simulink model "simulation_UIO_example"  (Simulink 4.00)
settings: Solver=VariableStepDiscrete  StartTime=0.0  StopTime=ts  RelTol=1e-3
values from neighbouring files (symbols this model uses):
  A = [0.9944 -0.1203 -0.4302    [UIO_example1.m]
  Ao = A - Ko*C    [UIO_example1.m]
  Auio = F    [UIO_example1.m]
  B = [0.4252 -0.0082 0.1813]'    [UIO_example1.m]
  Bo = [B Ko]    [UIO_example1.m]
  Buio = [T*B K]    [UIO_example1.m]
  C = eye(3)    [UIO_example1.m]
  Co = C    [UIO_example1.m]
  Cuio = C    [UIO_example1.m]
  D = zeros(3,3)    [UIO_example1.m]
  Do = zeros(3,4)    [UIO_example1.m]
  Duio = [zeros(3,1) H]    [UIO_example1.m]
  Tc = 0.1    [UIO_example1.m]
  x0 = [0.01 0.02 0.03]    [UIO_example1.m]

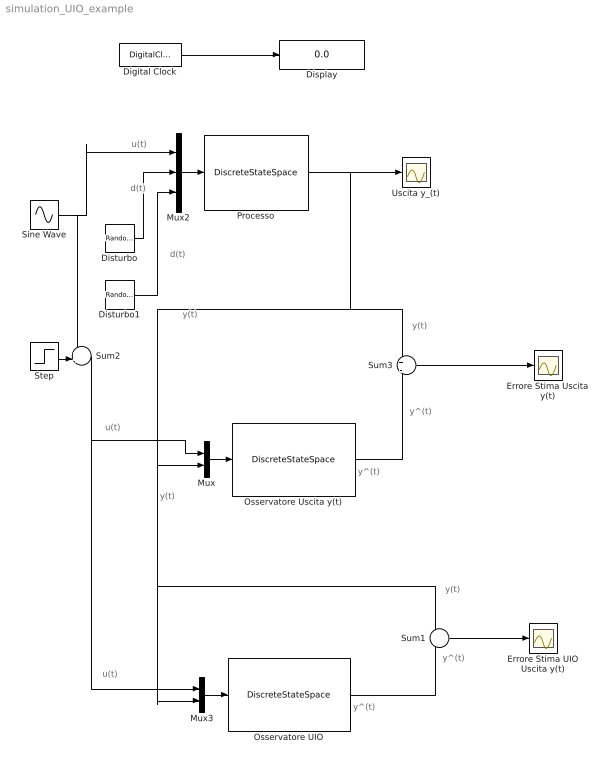
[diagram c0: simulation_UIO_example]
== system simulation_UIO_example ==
  note: d(t)
  note: u(t)
  note: y^(t)
  note: y(t)
  note: y^(t)
  note: y^(t)
  note: y^(t)
  note: y(t)
  note: d(t)
  note: u(t)
  note: u(t)
  note: y(t)
  note: y(t)
  Digital Clock : DigitalClock  SampleTime=Tc
  Display : Display
  Disturbo : RandomNumber  Mean=0  Variance=0.05  Seed=0  SampleTime=Tc
  Disturbo1 : RandomNumber  Mean=0  Variance=0.05  Seed=0  SampleTime=Tc
  Errore Stima Uscita y(t) : Scope
  Errore Stima UIO Uscita y(t) : Scope
  Mux : Mux  Inputs=2
  Mux2 : Mux  Inputs=3
  Mux3 : Mux  Inputs=2
  Osservatore UIO : DiscreteStateSpace  A=Auio  B=Buio  C=Cuio  D=Duio  X0=0  SampleTime=Tc  Realization=auto
  Osservatore Uscita y(t) : DiscreteStateSpace  A=Ao  B=Bo  C=Co  D=Do  X0=0  SampleTime=Tc  Realization=auto
  Processo : DiscreteStateSpace  A=A  B=[B E]  C=C  D=D  X0=x0  SampleTime=Tc  Realization=auto
  Sine Wave : Sin  SineType=Time-based  Amplitude=1  Bias=0  Frequency=1  Phase=0  Samples=10  SampleTime=Tc
  Step : Step  Time=25  Before=0  After=1  SampleTime=0
  Sum1 : Sum  Inputs=+|-  SaturateOnIntegerOverflow=on
  Sum2 : Sum  Inputs=++|  SaturateOnIntegerOverflow=on
  Sum3 : Sum  Inputs=+|-  SaturateOnIntegerOverflow=on
  Uscita y_(t) : Scope
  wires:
  Digital Clock/1 -> Display/1
  Mux2/1 -> Processo/1
  Sine Wave/1 -> Mux2/1, Sum2/1
  Processo/1 -> Sum3/1, Mux/2, Mux3/2, Sum1/1, Uscita y_(t)/1
  Disturbo/1 -> Mux2/2
  Mux/1 -> Osservatore Uscita y(t)/1
  Osservatore Uscita y(t)/1 -> Sum3/2
  Sum3/1 -> Errore Stima Uscita y(t)/1
  Mux3/1 -> Osservatore UIO/1
  Osservatore UIO/1 -> Sum1/2
  Sum1/1 -> Errore Stima UIO Uscita y(t)/1
  Disturbo1/1 -> Mux2/3
  Step/1 -> Sum2/2
  Sum2/1 -> Mux/1, Mux3/1
